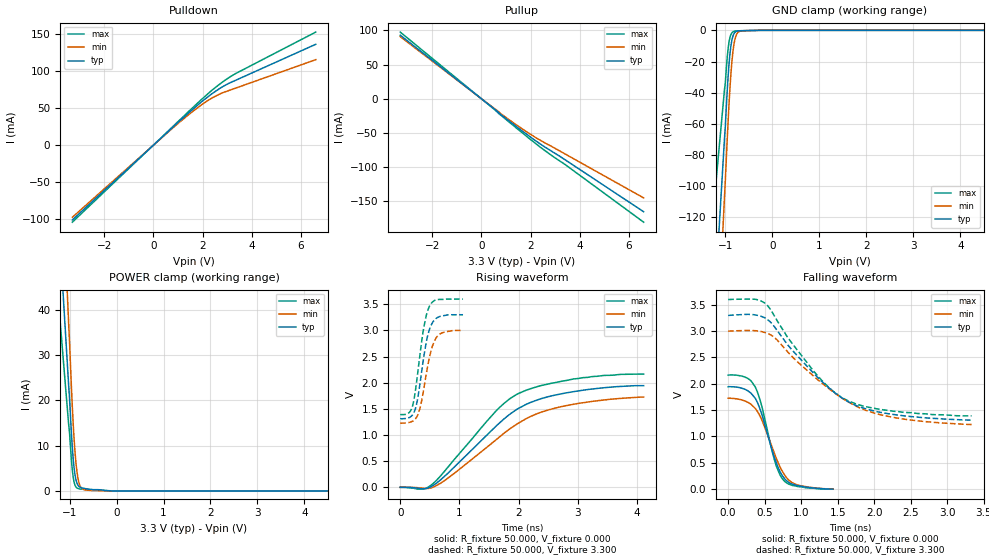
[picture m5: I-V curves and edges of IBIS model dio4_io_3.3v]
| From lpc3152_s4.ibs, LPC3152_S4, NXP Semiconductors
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[Model]   dio4_io_3.3v
Model_type I/O
Vinl=9.900E-01
Vinh=2.310E+00
Vref=0.000E+00
Rref=1.000E+06
Cref=2.500E-11
Vmeas=1.650E+00
C_comp   5.880E-13   5.740E-13   6.020E-13
[Voltage Range]   3.300E+00   3.000E+00   3.600E+00
[POWER Clamp Reference]   3.300E+00   3.000E+00   3.600E+00
[GND Clamp Reference]   0.000E+00   0.000E+00   0.000E+00
[Pullup Reference]   3.300E+00   3.000E+00   3.600E+00
[Pulldown Reference]   0.000E+00   0.000E+00   0.000E+00
[Temperature Range]   25   85   -40
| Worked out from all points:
|   slope of the pulldown table from 0 to 0.495 V, typ, clamps not added: 32.6 ohm
|   slope of the pullup table from 0 to 0.495 V, typ, clamps not added: 35.2 ohm
|   GND clamp passes 1 mA (typ) near -0.78 V on its own axis
|   POWER clamp passes 1 mA (typ) near -0.80 V on its own axis
|   rising waveform, R_fixture 50.000, V_fixture 0.000: 20-80 % time 1.16ns typ, 1.25ns min, 1.06ns max; typ from 0 V to 1.94 V
|   falling waveform, R_fixture 50.000, V_fixture 0.000: 20-80 % time 265ps typ, 301ps min, 234ps max; typ from 1.94 V to 0 V
|   rising waveform, R_fixture 50.000, V_fixture 3.300: 20-80 % time 168ps typ, 181ps min, 161ps max; typ from 1.31 V to 3.3 V
|   falling waveform, R_fixture 50.000, V_fixture 3.300: 20-80 % time 857ps typ, 953ps min, 773ps max; typ from 3.3 V to 1.31 V
[GND Clamp]
-3.3V     -1.222A    -1.527A    -786.6mA
-1.02V    -69.87mA   -107.5mA   -38.33mA
-1V       -60.93mA   -95.55mA   -33.25mA
-960mV    -38.31mA   -69.55mA   -17.09mA
-920mV    -20.65mA   -45.88mA   -7.064mA
-880mV    -9.463mA   -26.93mA   -2.544mA
-860mV    -6.062mA   -19.64mA   -1.529mA
-820mV    -2.307mA   -9.405mA   -657.8uA
-780mV    -899.5uA   -3.982mA   -405.8uA
-740mV    -445.7uA   -1.576mA   -313.4uA
-600mV    -222.8uA   -226.1uA   -251.4uA
6.6V      0A         0A         0A
[Power Clamp]
-3.3V     414.3mA    568mA      299.9mA
-1.02V    23.46mA    37.2mA     14.83mA
-1V       20.41mA    32.87mA    12.76mA
-960mV    12.73mA    22.86mA    6.822mA
-920mV    6.787mA    14.33mA    2.851mA
-880mV    3.297mA    8.086mA    1.171mA
-860mV    2.313mA    5.812mA    815.8uA
-820mV    1.237mA    2.743mA    533.5uA
-780mV    829.1uA    1.167mA    434.8uA
-720mV    633.3uA    433.5uA    373uA
-500mV    282uA      80.29uA    258.7uA
6.6V      0A         0A         0A
[Pullup]
-3.3V     92.86mA    90.84mA    97.47mA
60mV      -1.666mA   -1.651mA   -1.809mA
800mV     -23.53mA   -22.24mA   -24.35mA
1.88V     -53mA      -49.4mA    -56.3mA
2.66V     -72.43mA   -66.13mA   -77.89mA
3.46V     -90.65mA   -81.96mA   -97.72mA
6.6V      -165.3mA   -145.1mA   -180.6mA
[Pulldown]
-3.3V     -100.8mA   -97.23mA   -103.8mA
980mV     30.01mA    28.62mA    31.16mA
1.48V     44.88mA    42.38mA    46.91mA
2.16V     63.72mA    58.96mA    67.59mA
2.78V     78.09mA    70.1mA     84.35mA
3.34V     87.32mA    76.77mA    96.4mA
6.6V      135.9mA    115.1mA    152.3mA
[Rising Waveform]
R_fixture = 50.000
V_fixture = 0.000
V_fixture_min = 0.000
V_fixture_max = 0.000
|  time   V(typ)   V(min)   V(max)
0s        0V         0V         0V
380ps     -29.19mV   -17.04mV   -34.37mV
535ps     21.02mV    -5.43mV    53.27mV
805ps     269.5mV    175.4mV    385mV
1.615ns   1.168V     905.6mV    1.457V
2ns       1.512V     1.23V      1.796V
2.35ns    1.684V     1.425V     1.937V
2.74ns    1.792V     1.548V     2.032V
3.44ns    1.904V     1.67V      2.14V
4.11ns    1.944V     1.726V     2.165V
[Falling Waveform]
R_fixture = 50.000
V_fixture = 0.000
V_fixture_min = 0.000
V_fixture_max = 0.000
|  time   V(typ)   V(min)   V(max)
0s        1.944V     1.726V     2.165V
225ps     1.898V     1.676V     2.13V
370ps     1.727V     1.535V     1.944V
455ps     1.446V     1.332V     1.605V
645ps     553.8mV    636.5mV    503.4mV
705ps     347.3mV    438.8mV    286.8mV
765ps     212.2mV    286.7mV    161mV
850ps     112.4mV    149.2mV    85.14mV
950ps     67.74mV    79.89mV    50.04mV
1.435ns   0V         0V         0V
[Rising Waveform]
R_fixture = 50.000
V_fixture = 3.300
V_fixture_min = 3.000
V_fixture_max = 3.600
|  time   V(typ)   V(min)   V(max)
0s        1.309V     1.227V     1.391V
140ps     1.329V     1.239V     1.419V
210ps     1.388V     1.265V     1.565V
275ps     1.587V     1.338V     2.007V
335ps     1.995V     1.521V     2.554V
400ps     2.517V     1.899V     3.074V
500ps     3.041V     2.52V      3.477V
575ps     3.197V     2.792V     3.57V
665ps     3.265V     2.928V     3.593V
1.06ns    3.3V       3V         3.6V
[Falling Waveform]
R_fixture = 50.000
V_fixture = 3.300
V_fixture_min = 3.000
V_fixture_max = 3.600
|  time   V(typ)   V(min)   V(max)
0s        3.3V       3V         3.6V
375ps     3.306V     3.008V     3.604V
515ps     3.242V     2.969V     3.519V
635ps     3.082V     2.879V     3.285V
810ps     2.75V      2.615V     2.892V
1.205ns   2.152V     2.104V     2.186V
1.44ns    1.854V     1.843V     1.856V
1.635ns   1.667V     1.663V     1.682V
2.265ns   1.417V     1.361V     1.479V
3.335ns   1.309V     1.227V     1.391V
[Ramp]
dV/dt_r   1.1668E+00/1.1564E-09   1.0366E+00/1.2529E-09   1.2998E+00/1.0587E-09
dV/dt_f   1.1943E+00/8.5809E-10   1.0639E+00/9.5292E-10   1.3253E+00/7.7282E-10
R_load = 50
